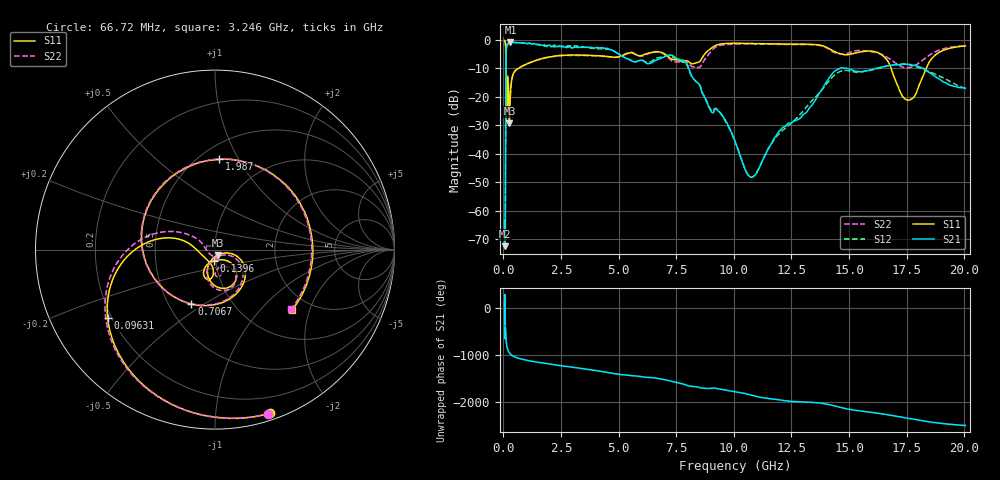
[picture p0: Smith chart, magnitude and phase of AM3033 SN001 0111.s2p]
# Hz S DB R 50
!freq MagS11 AngS11 MagS21 AngS21 MagS12 AngS12 MagS22 AngS22
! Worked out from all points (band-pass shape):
!   1601 points, 50 MHz to 20.05 GHz, reference 50 ohm
!   highest |S21| = -0.72 dB at 301.9 MHz (marker M1); lowest = -72.6 dB at 67.98 MHz (marker M2)
!   |S21| within 3 dB of the highest: 122.3 MHz to 4.764 GHz (4.641 GHz wide, 190 % of centre)
!   lowest |S11| = -29.2 dB at 257 MHz (marker M3), VSWR 1.07, Z = 51.4 - j3.21 ohm
!   |S11| at or under -10 dB: 103.7 MHz to 627.9 MHz (524.2 MHz wide, 143 % of centre); 16.83 GHz to 18.35 GHz (1.516 GHz wide, 8.62 % of centre)
!   |S22| runs from -28.6 to -0.1 dB; largest |S21 - S12| = 0.063
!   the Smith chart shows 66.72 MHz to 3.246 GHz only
!   S11 on the Smith chart (normalised r, x): 66.72 MHz: 0.06, -1.39; 96.31 MHz: 0.18, -0.28; 139.6 MHz: 0.98, -0.12; 706.7 MHz: 0.65, -0.44; 1.987 GHz: 0.62, +0.84; 3.246 GHz: 1.61, -1.53
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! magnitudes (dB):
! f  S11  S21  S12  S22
! 50 MHz  -0.1  -63.5  -64.1  -0.1
! 66.72 MHz  -0.3  -71.5  -70.0  -0.3
! 67.98 MHz  -0.4  -72.6  -70.3  -0.4
! 79.86 MHz  -0.7  -65.9  -65.7  -0.7
! 96.31 MHz  -3.0  -27.2  -27.2  -3.0
! 111.9 MHz  -22.5  -6.0  -6.0  -28.6
! 135.9 MHz  -21.4  -2.5  -2.5  -19.0
! 139.6 MHz  -24.0  -2.3  -2.3  -19.7
! 185.5 MHz  -13.2  -1.4  -1.4  -12.8
! 257 MHz  -29.2  -0.8  -0.8  -27.4
! 301.9 MHz  -18.6  -0.7  -0.7  -18.9
! 369.6 MHz  -13.5  -0.8  -0.8  -13.7
! 706.7 MHz  -9.6  -0.9  -1.0  -9.6
! 1.005 GHz  -8.5  -1.3  -1.1  -8.4
! 1.987 GHz  -6.0  -1.7  -2.2  -6.0
! 2.722 GHz  -5.3  -2.6  -2.2  -5.4
! 3.246 GHz  -5.3  -2.6  -2.2  -5.4
! 7.402 GHz  -6.9  -5.8  -6.3  -7.6
! 10.77 GHz  -1.2  -48.3  -48.3  -1.4
! 14.58 GHz  -4.7  -10.0  -11.2  -4.9
! 17.59 GHz  -21.1  -8.6  -8.6  -9.7
! 20.05 GHz  -2.1  -17.0  -17.0  -2.0
